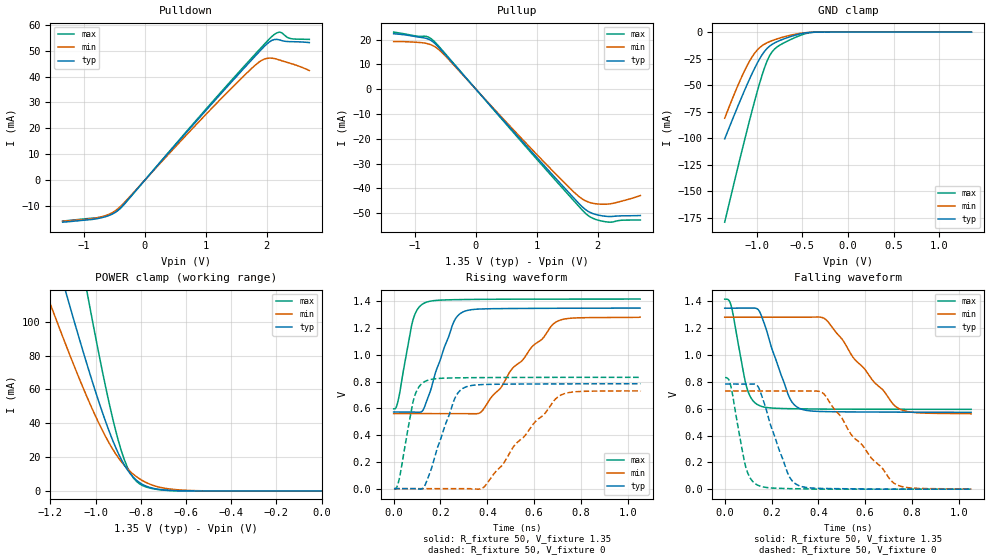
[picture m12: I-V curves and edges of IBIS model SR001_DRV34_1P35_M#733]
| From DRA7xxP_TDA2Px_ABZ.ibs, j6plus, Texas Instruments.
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| Model based on original model for DDR_DIFFIOPB_V
|   Sub model SR001_DRV34_1P35
[model]   SR001_DRV34_1P35_M#733
|[Description]  [1.35V-I/O-X-X]
|   , ,
|[Input Load]
|[Output Drive]
|Voltage   1.35V
|Mode   I/O
Model_type   I/O
Polarity   Non-Inverting
Enable   Active-Low
Vinl =  0.585
Vinh =  0.765
Cref =  15.0000pF
Rref =  100.0000M
Vref =  0V
Vmeas =  0.675
C_comp   2p   2p   2p
[Model Spec]
Vinl   0.585   0.55125   0.61875
Vinh   0.765   0.73125   0.79875
[Receiver Thresholds]
Tslew_ac = 5n
Vth = 0.675
Vth_max = 0.709
Vth_min = 0.608
Vinh_ac = 0.175
Vinh_dc = 0.1
Vinl_ac = -0.175
Vinl_dc = -0.1
[Temperature Range]   25   125   -40
[Voltage Range]   1.35   1.2825   1.4175
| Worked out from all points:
|   slope of the pulldown table from 0 to 0.203 V, typ, clamps not added: 36.8 ohm
|   slope of the pullup table from 0 to 0.203 V, typ, clamps not added: 36 ohm
|   GND clamp passes 1 mA (typ) near -0.48 V on its own axis
|   POWER clamp passes 1 mA (typ) near -0.72 V on its own axis
|   rising waveform, R_fixture 50, V_fixture 1.35: 20-80 % time 89ps typ, 215ps min, 51ps max; typ from 0.573 V to 1.35 V
|   rising waveform, R_fixture 50, V_fixture 0: 20-80 % time 88.5ps typ, 209ps min, 51.3ps max; typ from 0 V to 0.784 V
|   falling waveform, R_fixture 50, V_fixture 1.35: 20-80 % time 89.2ps typ, 199ps min, 52.9ps max; typ from 1.35 V to 0.573 V
|   falling waveform, R_fixture 50, V_fixture 0: 20-80 % time 89.3ps typ, 203ps min, 52.3ps max; typ from 0.784 V to 0 V
[POWER_clamp]
-1.35V    224.4mA    165.8mA    358.5mA
-1.214V   157mA      115.5mA    250.8mA
-1.132V   117.8mA    86.59mA    187.7mA
-1.118V   111.4mA    81.92mA    177.3mA
-1.036V   74.26mA    55.16mA    116.8mA
-954.5mV  40.7mA     31.91mA    61.06mA
-900mV    22.42mA    19.79mA    30.14mA
-859.1mV  12.48mA    13.09mA    13.96mA
-804.5mV  4.85mA     7.084mA    4.132mA
-736.4mV  1.313mA    2.9mA      1.073mA
-627.3mV  101.6uA    577.3uA    45.9uA
0V        75.63nA    322.4nA    418.5nA
[Pulldown]
-1.35V    -16.25mA   -15.93mA   -15.81mA
-736.4mV  -14.67mA   -14.31mA   -14.33mA
-531.8mV  -13.09mA   -12.54mA   -12.91mA
-409.1mV  -10.94mA   -10.36mA   -11.07mA
1.145V    30.69mA    28.89mA    31.23mA
1.718V    45.54mA    42.37mA    46.27mA
1.923V    50.72mA    46.33mA    51.51mA
2.086V    53.98mA    47.12mA    55.52mA
2.209V    54.19mA    46.41mA    57.19mA
2.25V     53.89mA    46.1mA     56.9mA
2.373V    53.5mA     45.23mA    54.8mA
2.7V      53.13mA    42.33mA    54.36mA
[Pullup]
-1.35V    22.33mA    19.2mA     23.01mA
-981.8mV  21.15mA    18.91mA    21.43mA
-818.2mV  20.5mA     18.48mA    21.31mA
-736.4mV  19.62mA    17.88mA    20.36mA
-613.6mV  16.97mA    16.06mA    17.42mA
1.064V    -29.25mA   -27.93mA   -29.99mA
1.555V    -42.46mA   -40.17mA   -43.52mA
1.759V    -47.7mA    -44.45mA   -49.03mA
1.923V    -50.14mA   -45.98mA   -52.07mA
2.127V    -51.21mA   -46.35mA   -53.42mA
2.291V    -51.16mA   -45.77mA   -53.24mA
2.7V      -50.91mA   -42.85mA   -52.71mA
[GND_clamp]
-1.35V    -100.7mA   -81.27mA   -179.3mA
-1.241V   -77.31mA   -57.61mA   -140mA
-1.132V   -54.83mA   -36.31mA   -101.6mA
-1.05V    -39.08mA   -23.36mA   -74mA
-968.2mV  -25.28mA   -14.71mA   -48.34mA
-913.6mV  -18.13mA   -11.32mA   -33.52mA
-859.1mV  -13.28mA   -9.024mA   -22.35mA
-831.8mV  -11.61mA   -8.091mA   -18.64mA
-777.3mV  -9.078mA   -6.444mA   -14.07mA
-531.8mV  -1.871mA   -1.307mA   -3.441mA
-368.2mV  -88.76uA   -111.2uA   -158uA
1.35V     75.63nA    385.5nA    349.4nA
[Ramp]
dV/dt_f 0.46669258/89.288181p 0.43374199/0.19960833n 0.49356657/52.942465p
dV/dt_r  0.4729597/88.946218p 0.44199207/0.21079013n 0.50180852/51.456668p
R_load = 50
[Rising Waveform]
R_fixture = 50
V_fixture = 1.35
V_fixture_min = 1.2825
V_fixture_max = 1.4175
0s        573.3mV    561.4mV    596.4mV
21.13ps   572.5mV    561.3mV    674.1mV
83.52ps   572.4mV    561.3mV    1.267V
133.5ps   618.2mV    561.3mV    1.39V
253.7ps   1.234V     561.2mV    1.413V
296.4ps   1.321V     560.5mV    1.414V
375ps     1.344V     575.6mV    1.415V
505.1ps   1.347V     894.3mV    1.417V
697.3ps   1.349V     1.25V      1.417V
1.053ns   1.35V      1.282V     1.417V
[Rising Waveform]
R_fixture = 50
V_fixture = 0
V_fixture_min = 0
V_fixture_max = 0
1.366ps   0V         0V         0V
24.7ps    0V         0V         78.08mV
87.57ps   0V         0V         680.5mV
136.3ps   34.79mV    0V         803.9mV
258.6ps   664mV      0V         828.1mV
303.5ps   756.6mV    0V         829.2mV
387.8ps   778.8mV    15.98mV    830.5mV
518.4ps   781.8mV    327.8mV    831.5mV
712.2ps   783.3mV    697.5mV    832mV
1.054ns   784.4mV    732.7mV    832.1mV
[Falling Waveform]
R_fixture = 50
V_fixture = 1.35
V_fixture_min = 1.2825
V_fixture_max = 1.4175
0s        1.35V      1.282V     1.417V
29.1ps    1.35V      1.283V     1.358V
96.42ps   1.35V      1.283V     745.8mV
147.5ps   1.329V     1.283V     624mV
272.4ps   699.6mV    1.283V     600.5mV
318.2ps   603.7mV    1.282V     599.2mV
433.4ps   578.4mV    1.263V     597.3mV
552.4ps   576.1mV    974.7mV    596.4mV
741.6ps   574.5mV    603.3mV    595.9mV
1.053ns   573.3mV    561.4mV    595.7mV
[Falling Waveform]
R_fixture = 50
V_fixture = 0
V_fixture_min = 0
V_fixture_max = 0
1.366ps   784.4mV    732.7mV    832.1mV
26.65ps   784.6mV    732.8mV    766.7mV
92.68ps   784mV      732.8mV    149.1mV
144.1ps   760.2mV    732.8mV    27.38mV
268.7ps   120.8mV    732.7mV    4.296mV
313.7ps   29.12mV    732.5mV    2.919mV
423.2ps   5.073mV    711.3mV    0V
542.2ps   2.597mV    403.3mV    0V
729.3ps   0V         38.01mV    0V
1.054ns   0V         0V         0V
